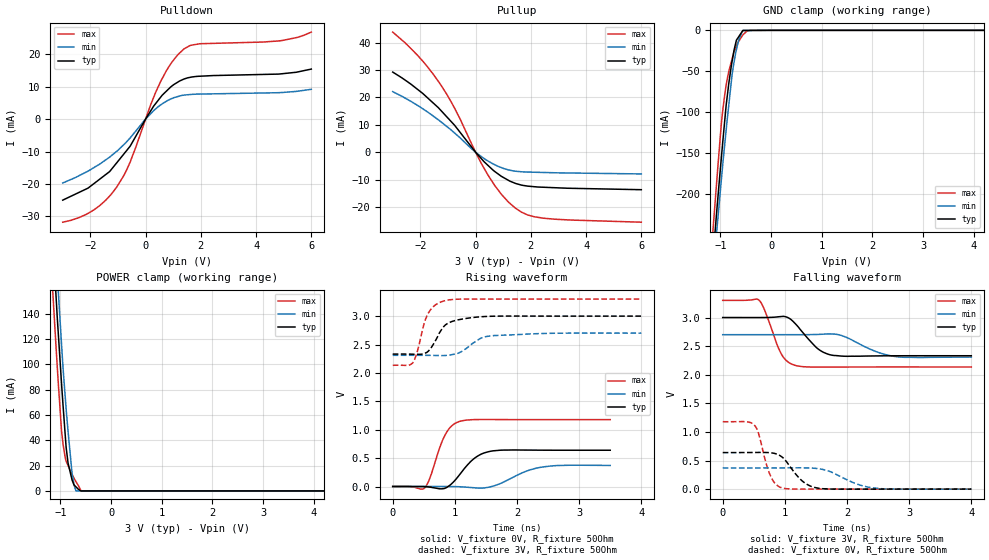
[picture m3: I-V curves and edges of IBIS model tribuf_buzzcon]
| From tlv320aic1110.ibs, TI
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|   tribuf_buzzcon Model
[Model]   tribuf_buzzcon
Model_type   3-state
Polarity   Non-Inverting
Enable   Active-Low
Vmeas = 1.5
Vref = 1.5
Cref = 15pF
Rref = 50
|   typ   min   max
|   (nom PVT)   (Fast PVT)   (slow PVT)
|Average
C_comp   2.597e-12   2.575e-12   2.598e-12
|ON state : BUFFER OUTPUT TURNED HIGH
|C_comp   2.597e-12   2.575e-12   2.598e-12
|OFF state: BUFFER IN HIGH IMPEDANCE
|C_comp   2.223e-12   2.215e-12   2.224e-12
| Where nom  PVT is Nominal Process,  3V,  65C
|   Fast PVT is Strong Process,   3.3V,  -40C
|   Slow PVT is Weak Process,   2.7V,  125C
[Voltage Range]   3   2.7   3.3
|Ambient Temperature   25   105   -40
|Junction Temperature
[Temperature Range]   65   125   -40
[Pullup Reference]   3   2.7   3.3
[Pulldown Reference]   0   0   0
[Power Clamp Reference]   3   2.7   3.3
[GND Clamp Reference]   0   0   0
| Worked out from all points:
|   slope of the pulldown table from 0 to 0.45 V, typ, clamps not added: 78.8 ohm
|   slope of the pullup table from 0 to 0.45 V, typ, clamps not added: 93.2 ohm
|   GND clamp passes 1 mA (typ) near -0.57 V on its own axis
|   POWER clamp passes 1 mA (typ) near -0.63 V on its own axis
|   falling waveform, V_fixture 3V, R_fixture 50Ohm: 20-80 % time 328ps typ, 458ps min, 244ps max; typ from 3 V to 2.33 V
|   rising waveform, V_fixture 0V, R_fixture 50Ohm: 20-80 % time 316ps typ, 445ps min, 234ps max; typ from 0 V to 0.638 V
|   rising waveform, V_fixture 3V, R_fixture 50Ohm: 20-80 % time 245ps typ, 319ps min, 188ps max; typ from 2.33 V to 3 V
|   falling waveform, V_fixture 0V, R_fixture 50Ohm: 20-80 % time 293ps typ, 448ps min, 184ps max; typ from 0.639 V to 0 V
[Pulldown]
|   Voltage   I(typ)   I(min)   I(max)
-3V       -24.97mA   -19.69mA   -31.76mA
-1.885V   -19.97mA   -15.02mA   -28.05mA
-1.299V   -16.15mA   -11.7mA    -23.67mA
-1.05V    -13.52mA   -9.964mA   -21mA
-564.6mV  -8.413mA   -5.85mA    -13.36mA
181.2mV   2.476mA    1.61mA     4.334mA
534.3mV   6.63mA     4.304mA    11.39mA
956.7mV   10.21mA    6.352mA    17.58mA
1.392V    12.35mA    7.395mA    21.63mA
1.976V    13.21mA    7.712mA    23.22mA
4.933V    13.96mA    8.188mA    24.19mA
6V        15.41mA    9.18mA     26.8mA
[GND Clamp]
-3V       -1.869A    -1.8A      -1.958A
-1.152V   -282.3mA   -302.9mA   -249.3mA
-1.089V   -234.5mA   -258.1mA   -198.1mA
-1.065V   -216.1mA   -240.9mA   -179mA
-980.4mV  -155.5mA   -182.5mA   -113.5mA
-950.7mV  -135mA     -162.4mA   -96.55mA
-882mV    -89.48mA   -119.3mA   -65.76mA
-783mV    -42.85mA   -62.06mA   -38.18mA
-684mV    -12.1mA    -23.67mA   -18.79mA
-554.7mV  -272.3uA   0A         -5.459mA
-410.7mV  -201uA     0A         0A
6V        0A         0A         0A
[Pullup]
|   Voltage   I(typ)   I(min)   I(max)
-3V       29.24mA    22.1mA     43.83mA
-2.116V   23.05mA    17.17mA    35.53mA
-1.357V   16.32mA    11.89mA    25.99mA
-1.036V   12.84mA    9.338mA    21.01mA
-759.3mV  9.819mA    6.991mA    16.06mA
49.2mV    -560uA     -388.3uA   -995.2uA
448.5mV   -4.816mA   -3.218mA   -8.348mA
943.5mV   -8.865mA   -5.663mA   -15.48mA
1.432V    -11.34mA   -6.926mA   -20.35mA
1.887V    -12.39mA   -7.258mA   -22.91mA
2.481V    -12.8mA    -7.41mA    -24.12mA
6V        -13.69mA   -7.936mA   -25.55mA
[POWER Clamp]
-3V       1.719A     1.684A     1.817A
-1.152V   200.3mA    232.8mA    158.5mA
-1.132V   185.9mA    218.4mA    144.2mA
-1.066V   139.8mA    174.2mA    100.5mA
-1.04V    123.2mA    156.4mA    83.97mA
-977.1mV  84.49mA    115.5mA    47.25mA
-885mV    33.78mA    63.81mA    23.24mA
-849mV    22mA       47.12mA    20.03mA
-769.8mV  8.602mA    13.87mA    13.05mA
-693.3mV  3.22mA     0A         7.364mA
-591mV    0A         0A         0A
6V        0A         0A         0A
[Ramp]
R_load = 50
|   typ   min   max
dV/dt_r   0.383292/3.16127e-10   0.222096/4.44182e-10   0.706871/2.34505e-10
dV/dt_f   0.401381/3.28278e-10   0.234071/4.5597e-10   0.699295/2.44285e-10
[Falling Waveform]
V_fixture = 3V
V_fixture_min = 2.7V
V_fixture_max = 3.3V
R_fixture = 50Ohm
|   Time   V(typ)   V(min)   V(max)
0s        3V         2.7V       3.3V
575ps     3V         2.7V       3.311V
675ps     3V         2.7V       3.127V
950ps     3.018V     2.7V       2.349V
1.05ns    2.999V     2.7V       2.224V
1.175ns   2.885V     2.7V       2.161V
1.525ns   2.459V     2.704V     2.133V
1.75ns    2.343V     2.713V     2.134V
2.75ns    2.331V     2.322V     2.135V
4ns       2.332V     2.309V     2.135V
[Rising Waveform]
V_fixture = 0V
V_fixture_min = 0V
V_fixture_max = 0V
R_fixture = 50Ohm
|   Time   V(typ)   V(min)   V(max)
0s        909.1pV    2.503nV    219pV
525ps     -3.108mV   91.22uV    -12.41mV
600ps     -11.26mV   123.7uV    154.2mV
775ps     -41.26mV   333.5uV    739.9mV
850ps     -26.73mV   128uV      922.2mV
1.075ns   206.7mV    -4.622mV   1.145V
1.325ns   504.8mV    -23.27mV   1.178V
1.6ns     625.3mV    2.333mV    1.179V
2.4ns     639.4mV    341.6mV    1.177V
3.5ns     638.4mV    370.7mV    1.177V
[Rising Waveform]
V_fixture = 3V
V_fixture_min = 2.7V
V_fixture_max = 3.3V
R_fixture = 50Ohm
|   Time   V(typ)   V(min)   V(max)
0s        2.331V     2.31V      2.135V
325ps     2.329V     2.31V      2.179V
400ps     2.327V     2.31V      2.392V
550ps     2.362V     2.309V     3.002V
650ps     2.497V     2.308V     3.163V
825ps     2.821V     2.305V     3.267V
1.05ns    2.934V     2.345V     3.298V
1.4ns     2.987V     2.601V     3.3V
1.6ns     2.998V     2.654V     3.299V
4ns       3V         2.7V       3.3V
[Falling Waveform]
V_fixture = 0V
V_fixture_min = 0V
V_fixture_max = 0V
R_fixture = 50Ohm
|   Time   V(typ)   V(min)   V(max)
0s        638.8mV    370.2mV    1.178V
500ps     640.5mV    370.1mV    1.129V
575ps     641.3mV    370.2mV    979.6mV
700ps     640.2mV    370.4mV    445.5mV
775ps     634.7mV    370.6mV    217.8mV
975ps     542.8mV    371.3mV    16.07mV
1.275ns   146.5mV    372.1mV    -200.7uV
1.55ns    14.13mV    355.9mV    59.93uV
2.4ns     -209.2uV   24.31mV    429.9uV
4ns       164.2uV    114.9uV    256.8uV
